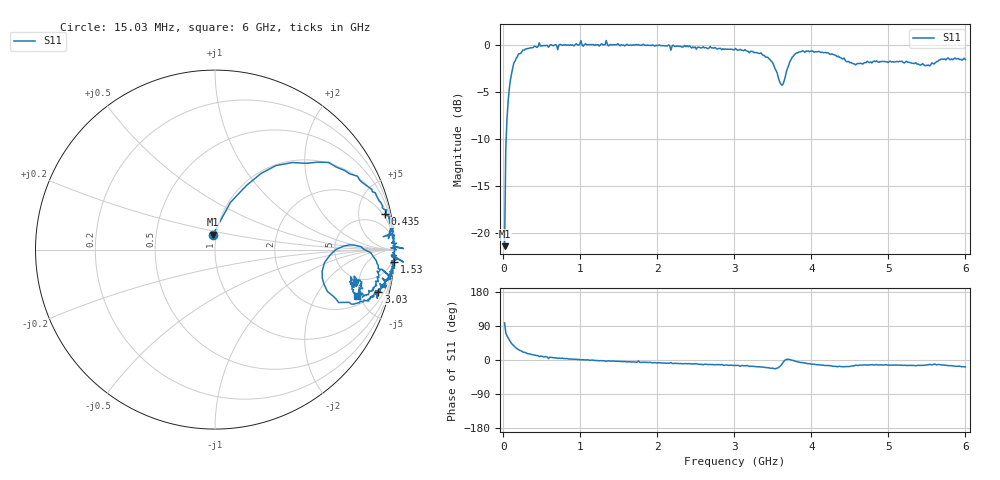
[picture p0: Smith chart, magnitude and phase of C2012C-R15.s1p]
!	Network	Analyzer	HP8753E.07.74:	Oct	30	2002	Serial	No.	JP38451487
!	Hewlett-Packard
!	7	Sep	2009	12:15:19
!	Frequency	S11
#	HZ	S	RI	R	50
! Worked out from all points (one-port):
!   400 points, 15.03 MHz to 6 GHz, reference 50 ohm
!   lowest |S11| = -21.4 dB at 15.03 MHz (marker M1), VSWR 1.19, Z = 48.2 + j8.16 ohm
!   |S11| at or under -10 dB: start of sweep to 35.55 MHz
!   S11 on the Smith chart (normalised r, x): 15.03 MHz: 0.96, +0.16; 435 MHz: 1.59, +9.44; 1.53 GHz: 0, -30; 3.03 GHz: 1.86, -7.45; 6 GHz: 2.79, -4.68
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1.502992e7  -0.0117 0.0841
3.002985e7  0.0862 0.263
6.00297e7  0.256 0.424
9.002955e7  0.431 0.485
1.95029e8  0.794 0.409
4.350278e8  0.946 0.197
5.550272e8  0.977 0.158
5.850271e8  0.966 0.0613
6.00027e8  0.983 0.124
7.650262e8  0.988 0.0844
1.005025e9  1.05 0.00592
1.245024e9  0.982 -0.0328
1.335023e9  1.05 -0.069
1.515022e9  0.984 -0.0634
1.530022e9  0.997 -0.0664
2.265019e9  0.971 -0.154
3.015015e9  0.924 -0.238
3.030015e9  0.91 -0.234
3.345013e9  0.857 -0.286
3.525012e9  0.689 -0.295
3.615012e9  0.597 -0.12
3.675012e9  0.719 0.0199
3.765011e9  0.868 -0.0177
4.06501e9  0.894 -0.199
4.515007e9  0.772 -0.224
5.265004e9  0.78 -0.202
5.595002e9  0.775 -0.148
6e9  0.791 -0.258
